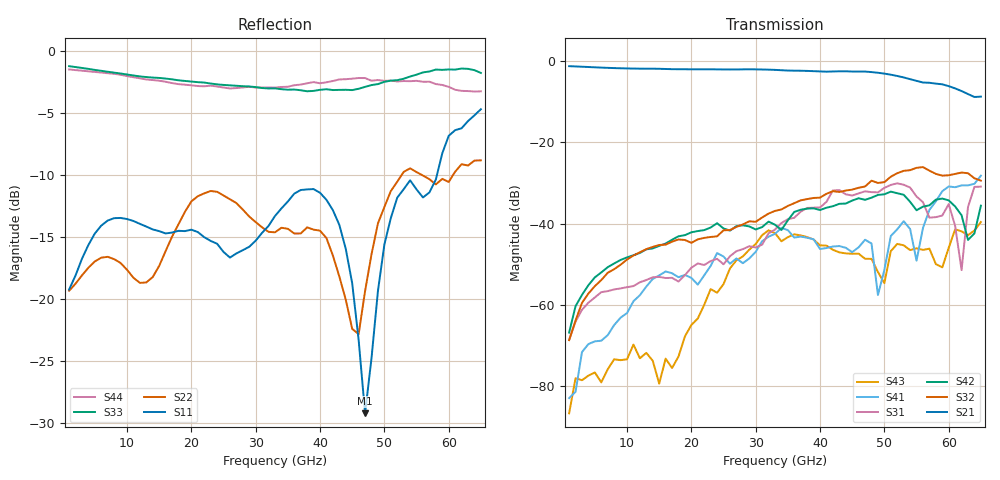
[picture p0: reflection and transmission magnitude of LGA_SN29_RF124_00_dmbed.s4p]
! Created Thu Nov 10 13:45:35 2022
# hz S ma R 50
! 4 Port Network Data from SP1.SP block
! freq  magS11  angS11  magS12  angS12  magS13  angS13  magS14  angS14
!  magS21  angS21  magS22  angS22  magS23  angS23  magS24  angS24
!  magS31  angS31  magS32  angS32  magS33  angS33  magS34  angS34
!  magS41  angS41  magS42  angS42  magS43  angS43  magS44  angS44
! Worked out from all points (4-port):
!   65 points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, 1 GHz to 65 GHz, reference 50 ohm
!   strongest paths, dB at 1 GHz, 17 GHz, 33 GHz, 49 GHz, 65 GHz:
!     S21: -1.3, -2.0, -2.2, -2.9, -8.8
!     S32: -68.7, -44.4, -36.9, -30.0, -29.4
!     S42: -66.8, -44.0, -40.3, -33.0, -35.6
!     S31: -68.6, -53.3, -41.5, -32.3, -30.9
!     S41: -82.9, -52.2, -42.5, -57.6, -28.2
!     S43: -86.7, -75.5, -42.3, -51.9, -39.6
!   lowest |S11| = -29.2 dB at 47 GHz (marker M1), VSWR 1.07, Z = 52.5 + j2.51 ohm
!   |S11| at or under -10 dB: start of sweep to 58.18 GHz
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1e9  0.109 -30.8  0.8622 -13.2  0.000375 66.9  0.0001725 73.4
     0.8617 -13.2  0.1078 -27.7  0.0003651 83.2  0.0005797 65.1
     0.0003718 69.3  0.0003683 70.9  0.865 169.8  0.0001025 55.3
     7.144e-05 27.1  0.0004567 69.7  4.646e-05 -140.4  0.8393 171.3
1.4e10  0.1903 -173.7  0.8027 -172.7  0.002088 -72.6  0.002018 20.8
        0.8025 -172.6  0.1224 -175.0  0.005219 -9.2  0.004901 -79.9
        0.002183 -68.5  0.005162 -10.2  0.7782 43.9  0.00022 -50.1
        0.002084 20.2  0.00495 -79.9  0.0002055 -38.1  0.7606 56.6
2.9e10  0.162 38.0  0.7887 1.6  0.005186 133.4  0.003629 177.3
        0.7888 1.6  0.2144 87.4  0.01058 153.8  0.009255 80.1
        0.005267 133.8  0.01067 156.0  0.7165 -122.1  0.004742 100.3
        0.00372 176.1  0.009233 80.6  0.004774 103.2  0.7149 -112.8
3.7e10  0.2743 -112.4  0.7572 -101.8  0.014 52.8  0.006349 30.4
        0.7572 -101.7  0.1833 71.0  0.01877 55.4  0.01469 1.4
        0.01403 53.1  0.01931 55.9  0.6918 144.6  0.007028 -34.1
        0.006922 32.4  0.01481 3.2  0.007152 -34.7  0.7294 168.3
4.7e10  0.03458 43.6  0.74 122.9  0.02531 -77.6  0.006096 100.6
        0.7398 122.9  0.1074 96.4  0.02861 -52.2  0.0203 -117.6
        0.02492 -76.6  0.0286 -53.1  0.714 37.5  0.004071 167.1
        0.006328 97.2  0.01959 -116.6  0.00369 155.1  0.7746 73.3
6.2e10  0.4862 162.1  0.426 -92.8  0.003286 77.7  0.03147 -67.7
        0.4262 -92.6  0.3485 -157.0  0.0404 86.3  0.0131 36.2
        0.002684 26.8  0.04241 87.0  0.8462 -118.7  0.008665 -90.7
        0.02948 -68.9  0.01265 33.0  0.008022 -91.5  0.688 -82.5
6.5e10  0.5803 144.7  0.3626 -126.8  0.02903 154.2  0.0404 -104.8
        0.3639 -126.7  0.3612 156.3  0.03168 42.3  0.01597 67.7
        0.02846 155.2  0.03371 45.8  0.8125 -140.3  0.01055 156.3
        0.03885 -107.2  0.0166 68.9  0.01044 146.8  0.6851 -126.2
